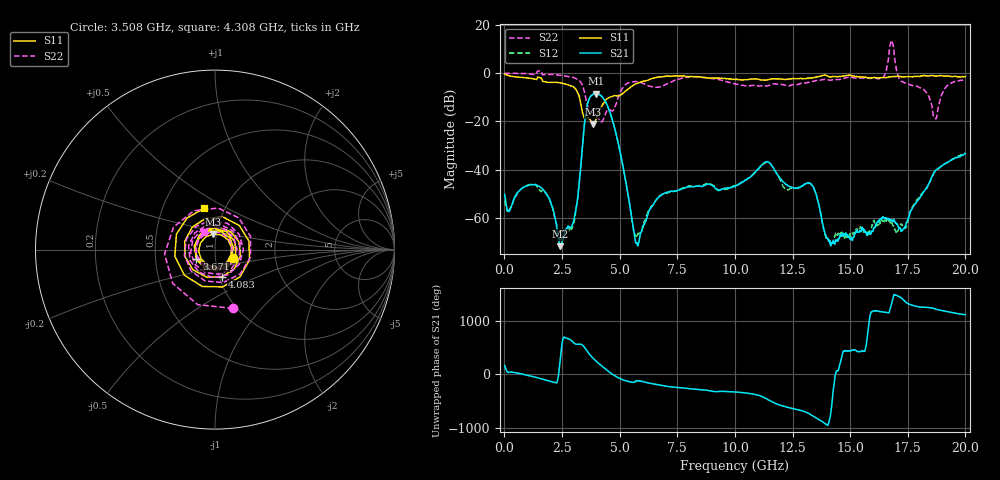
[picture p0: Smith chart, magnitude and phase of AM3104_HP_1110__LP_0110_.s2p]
!Created with skrf (http://scikit-rf.org).
# Hz S RI R 50.0
!freq ReS11 ImS11 ReS21 ImS21 ReS12 ImS12 ReS22 ImS22
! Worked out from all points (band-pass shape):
!   1601 points, 10 MHz to 20 GHz, reference 50 ohm
!   highest |S21| = -8.49 dB at 3.983 GHz (marker M1); lowest = -71.7 dB at 2.409 GHz (marker M2)
!   |S21| within 3 dB of the highest: 3.645 GHz to 4.364 GHz (719.4 MHz wide, 18 % of centre)
!   lowest |S11| = -21.2 dB at 3.858 GHz (marker M3), VSWR 1.19, Z = 48.4 + j8.48 ohm
!   |S11| at or under -10 dB: 3.255 GHz to 4.571 GHz (1.316 GHz wide, 33.6 % of centre)
!   |S22| runs from -20.3 to 13.5 dB; largest |S21 - S12| = 0.027
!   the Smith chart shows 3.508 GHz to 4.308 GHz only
!   S11 on the Smith chart (normalised r, x): 3.508 GHz: 1.22, -0.12; 3.671 GHz: 0.81, -0.08; 4.083 GHz: 1.03, -0.32; 4.308 GHz: 0.80, +0.39
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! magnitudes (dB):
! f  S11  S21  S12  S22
! 10 MHz  -0.4  -50.2  -52.7  0.0
! 1.584 GHz  -2.0  -47.4  -48.9  0.9
! 2.409 GHz  -4.0  -71.7  -69.2  -0.9
! 2.996 GHz  -5.7  -61.5  -61.9  -1.8
! 3.346 GHz  -14.3  -34.9  -34.9  -4.2
! 3.508 GHz  -18.9  -18.2  -18.3  -9.3
! 3.671 GHz  -18.8  -10.8  -10.9  -15.0
! 3.858 GHz  -21.2  -8.7  -8.7  -16.8
! 3.983 GHz  -18.9  -8.5  -8.5  -17.4
! 4.083 GHz  -16.1  -8.7  -8.7  -18.6
! 4.308 GHz  -12.5  -10.6  -10.6  -18.8
! 5.732 GHz  -4.3  -70.4  -66.8  -3.5
! 6.682 GHz  -1.6  -51.5  -51.3  -5.8
! 10.01 GHz  -2.7  -47.1  -46.7  -4.5
! 11.38 GHz  -2.9  -36.7  -36.9  -5.3
! 13.34 GHz  -2.1  -46.4  -46.3  -3.6
! 14.17 GHz  -1.5  -71.3  -71.6  -2.9
! 16.36 GHz  -1.9  -60.1  -60.4  -2.3
! 16.68 GHz  -1.6  -60.7  -61.2  7.1
! 17.3 GHz  -1.6  -64.6  -64.0  -3.7
! 18.69 GHz  -1.2  -40.5  -40.7  -18.8
! 20 GHz  -1.4  -33.3  -33.2  -2.6
